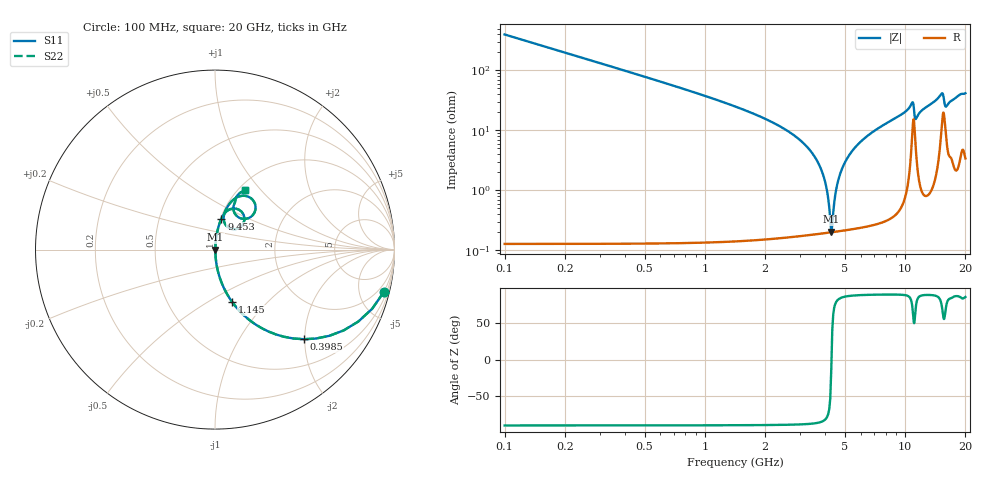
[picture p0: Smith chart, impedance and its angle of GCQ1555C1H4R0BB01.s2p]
!Murata Part Number: GCQ1555C1H4R0BB01
!These Parameters are Measured in Series Mode Connection
!Data Generated on Jan 08, 2026
!  o--ll--o
!Port1  Port2
!  o------o
!Operation Temp=25[degC], DC Bias Voltage=0[V]
!Freq. Start=100[MHz] Stop=20[GHz] 401[Steps]
# Hz S RI R 50
!Freq.(Hz) S11(Real) S11(Imag) S21(Real) S21(Imag) S12(Real) S12(Imag) S22(Real) S22(Imag)
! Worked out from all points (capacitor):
!   401 points, 100 MHz to 20 GHz, reference 50 ohm
!   read as one part in series: C = 4 pF near 199.5 MHz
!   lowest |Z| = 204 mohm at 4.279 GHz (marker M1)
!   series resonance near 4.289 GHz, so ESL is about 340 pH
!   S11 on the Smith chart (normalised r, x): 100 MHz: 1.00, -7.95; 398.5 MHz: 1.00, -1.98; 1.145 GHz: 1.00, -0.65; 9.453 GHz: 1.01, +0.36; 20 GHz: 1.07, +0.83
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1e8  0.9405 -0.2365  0.0595 0.2365  0.0595 0.2365  0.9405 -0.2365
3.985e8  0.4949 -0.4993  0.5051 0.4993  0.5051 0.4993  0.4949 -0.4993
6.97e8  0.2366 -0.4238  0.7634 0.4238  0.7634 0.4238  0.2366 -0.4238
1.14475e9  0.0954 -0.2917  0.9046 0.2917  0.9046 0.2917  0.0954 -0.2917
3.43325e9  0.00355 -0.0416  0.9965 0.0416  0.9965 0.0416  0.00355 -0.0416
3.93075e9  0.00218 -0.0162  0.9978 0.0162  0.9978 0.0162  0.00218 -0.0162
4.279e9  0.00199 -0.000442  0.998 0.000442  0.998 0.000442  0.00199 -0.000442
4.3785e9  0.00202 0.00384  0.998 -0.00384  0.998 -0.00384  0.00202 0.00384
4.478e9  0.00209 0.00803  0.9979 -0.00803  0.9979 -0.00803  0.00209 0.00803
4.62725e9  0.00226 0.0142  0.9977 -0.0142  0.9977 -0.0142  0.00226 0.0142
5.02525e9  0.00303 0.0297  0.997 -0.0297  0.997 -0.0297  0.00303 0.0297
5.72175e9  0.00531 0.0547  0.9947 -0.0547  0.9947 -0.0547  0.00531 0.0547
6.7665e9  0.0105 0.0888  0.9895 -0.0888  0.9895 -0.0888  0.0105 0.0888
9.453e9  0.0354 0.1717  0.9646 -0.1717  0.9646 -0.1717  0.0354 0.1717
1.005e10  0.0478 0.1945  0.9522 -0.1945  0.9522 -0.1945  0.0478 0.1945
1.0846e10  0.1326 0.2227  0.8674 -0.2227  0.8674 -0.2227  0.1326 0.2227
1.129375e10  0.0679 0.128  0.9321 -0.128  0.9321 -0.128  0.0679 0.128
1.338325e10  0.0765 0.2492  0.9235 -0.2492  0.9235 -0.2492  0.0765 0.2492
1.5423e10  0.2262 0.2388  0.7738 -0.2388  0.7738 -0.2388  0.2262 0.2388
1.587075e10  0.1352 0.1776  0.8648 -0.1776  0.8648 -0.1776  0.1352 0.1776
1.67165e10  0.1078 0.2548  0.8922 -0.2548  0.8922 -0.2548  0.1078 0.2548
2e10  0.1666 0.3339  0.8334 -0.3339  0.8334 -0.3339  0.1666 0.3339
